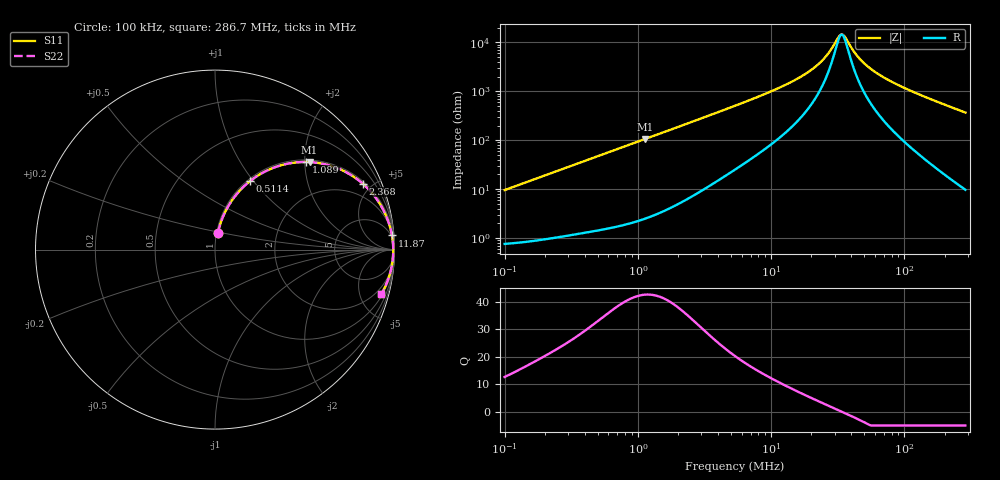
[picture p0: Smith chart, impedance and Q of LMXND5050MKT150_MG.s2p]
! LMXND5050MKT150_MG  S-PARAMETER MODEL  ( General Type )
! Model Generated by TAIYO YUDEN Corporation (https://www.yuden.co.jp/en/)
! Version 1.0
! TAIYO YUDEN Control No. 191023NI43SB-FBB
! Copyright(c) 2019 TAIYO YUDEN CO.,LTD. All Rights Reserved.
! Product Description (link to TY-COMPAS)
! https://ds.yuden.co.jp/TYCOMPAS/or/detail?pn=LMXND5050MKT150MMG&u=M
! Products Name : Inductors
! Characteristics :
!  Inductance : 15 uH , SRF(min) : 22 MHz , DC Resistance(max) : 0.804 Ohm
!  Rated Current : Saturation :1200 mA , Temp Rise : 640 mA (40 degC)
!  Case Size : 4.9 x 4.9 / 0.193 x 0.193 [mm/inch] , Thickness : 1.2 / 0.047 [mm/inch]
!  (Conditions: Temperature = 25 degC , DC Bias Current/Voltage = 0A / 0V)
! External Node Assignments :
!  1  o---GGG---o  2
! GND o---------o GND
! Frequency Range : 0.1MHz  -  286.687601MHz  [ 402 STEP ]
# MHz S RI R 50
! Freq[MHz].  S11 Real  S11 Imag  S21 Real  S21 Imag  S12 Real  S12 Imag  S22 Real  S22 Imag
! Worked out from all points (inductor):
!   401 points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, 100 kHz to 286.7 MHz, reference 50 ohm
!   read as one part in series: L = 15.1 uH near 104.1 kHz
!   highest Q = 42.5 at 1.134 MHz (marker M1), where L = 14.8 uH
!   self-resonance near 33.41 MHz
!   S11 on the Smith chart (normalised r, x): 100 kHz: 1.02, +0.19; 511.4 kHz: 1.03, +0.96; 1.089 MHz: 1.05, +2.03; 2.368 MHz: 1.13, +4.42; 11.87 MHz: 3, +25; 286.7 MHz: 1.19, -7.36
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0.1  0.0163 0.093  0.9837 -0.093  0.9837 -0.093  0.0163 0.093
0.217319  0.049 0.1936  0.951 -0.1936  0.951 -0.1936  0.049 0.1936
0.379416  0.1212 0.3093  0.8788 -0.3093  0.8788 -0.3093  0.1212 0.3093
0.51141  0.1938 0.3806  0.8062 -0.3806  0.8062 -0.3806  0.1938 0.3806
0.776753  0.3484 0.464  0.6516 -0.464  0.6516 -0.464  0.3484 0.464
1.089489  0.5078 0.4883  0.4922 -0.4883  0.4922 -0.4883  0.5078 0.4883
1.13373  0.5272 0.4876  0.4728 -0.4876  0.4728 -0.4876  0.5272 0.4876
1.439567  0.6398 0.4682  0.3602 -0.4682  0.3602 -0.4682  0.6398 0.4682
2.367664  0.823 0.3676  0.177 -0.3676  0.177 -0.3676  0.823 0.3676
5.354322  0.9539 0.1864  0.0461 -0.1864  0.0461 -0.1864  0.9539 0.1864
11.86985  0.9858 0.0791  0.0142 -0.0791  0.0142 -0.0791  0.9858 0.0791
20.31517  0.9917 0.0341  0.00828 -0.0341  0.00828 -0.0341  0.9917 0.0341
25.28711  0.9927 0.019  0.00731 -0.019  0.00731 -0.019  0.9927 0.019
32.10861  0.9932 0.00341  0.00684 -0.00341  0.00684 -0.00341  0.9932 0.00341
34.08411  0.9932 -0.000422  0.00681 0.000422  0.00681 0.000422  0.9932 -0.000422
36.18117  0.9932 -0.00426  0.0068 0.00426  0.0068 0.00426  0.9932 -0.00426
42.42587  0.993 -0.0146  0.00696 0.0146  0.00696 0.0146  0.993 -0.0146
48.76805  0.9927 -0.0239  0.00729 0.0239  0.00729 0.0239  0.9927 -0.0239
59.50735  0.9918 -0.0381  0.00816 0.0381  0.00816 0.0381  0.9918 -0.0381
77.07906  0.9898 -0.0588  0.0102 0.0588  0.0102 0.0588  0.9898 -0.0588
134.5721  0.9791 -0.1178  0.0209 0.1178  0.0209 0.1178  0.9791 -0.1178
286.6876  0.9255 -0.2497  0.0745 0.2497  0.0745 0.2497  0.9255 -0.2497
